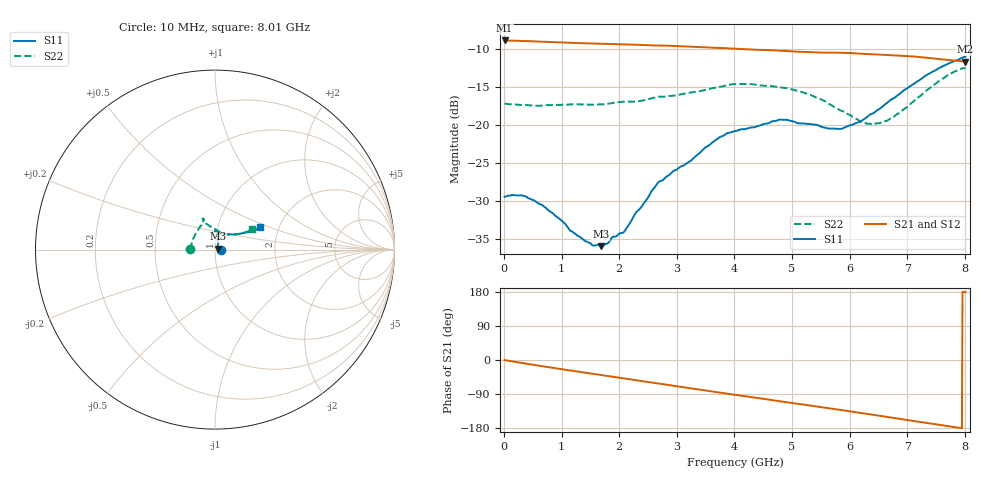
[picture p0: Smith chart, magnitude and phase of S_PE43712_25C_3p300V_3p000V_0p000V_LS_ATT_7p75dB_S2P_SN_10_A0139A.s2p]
! DEVICE ID: PE43712
! File Path: z:\PE43713\PE43713_CHAR_NOM_04292014\AMB\3p300\LS_ATT_7p75dB\PE43713_AMB_3p300V_3p000V_0p000V_LS_ATT_7p75dB_S2P_SN_10_A0139A.s2p
! Serial: 10
! Lot: A0139A
! Temp: 25C
! VDD: 3.300
! VSS: 0.000
! Control_Hi: 3.000
! Control_Lo: 0.000
! Attenuation Step: 7.75dB
! Port 1: RF1
! Port 2: RF2
! ThroughPath:1-2
! IDD: 0.0001474223
! ISS: -2.092e-007
#  Hz  S  RI  R  50
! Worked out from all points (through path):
!   801 points, 10 MHz to 8.01 GHz, reference 50 ohm
!   highest |S21| = -8.90 dB at 10 MHz (marker M1); lowest = -11.7 dB at 8.01 GHz (marker M2)
!   group delay of S21, straight-line fit = 62.2 ps
!   lowest |S11| = -35.9 dB at 1.68 GHz (marker M3), VSWR 1.03, Z = 51.5 + j0.548 ohm
!   |S11| at or under -10 dB: start of sweep to end of sweep
!   |S22| runs from -20.0 to -12.5 dB; largest |S21 - S12| = 0.0012
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1e7  0.0337 0.00011  0.3588 -0.0019  0.3588 -0.00189  -0.138 0.000826
3e8  0.0341 -0.00435  0.3531 -0.0474  0.353 -0.0474  -0.1345 0.0138
5.1e8  0.0315 -0.00604  0.3452 -0.0782  0.3452 -0.0781  -0.1319 0.0223
6.9e8  0.0284 -0.00621  0.3364 -0.1029  0.3364 -0.103  -0.1305 0.031
1.35e9  0.0179 -0.00129  0.2916 -0.1828  0.2917 -0.1829  -0.1227 0.059
1.55e9  0.0159 0.00231  0.2749 -0.2041  0.2749 -0.2041  -0.117 0.0688
1.68e9  0.015 0.00532  0.2634 -0.217  0.2634 -0.2171  -0.1143 0.0748
2.09e9  0.0133 0.0148  0.2231 -0.254  0.2231 -0.2539  -0.106 0.0942
2.68e9  0.0183 0.0379  0.1561 -0.293  0.1561 -0.293  -0.0822 0.1293
3.24e9  0.014 0.0563  0.0863 -0.3149  0.0864 -0.3149  -0.0707 0.1467
3.72e9  0.0117 0.081  0.0262 -0.3193  0.0259 -0.3193  -0.0657 0.1646
4.01e9  0.00784 0.0908  -0.00994 -0.3168  -0.00995 -0.3168  -0.0683 0.1723
4.79e9  0.00248 0.1083  -0.0993 -0.2909  -0.0993 -0.2911  -0.0638 0.1653
5.35e9  0.0139 0.0999  -0.1542 -0.2579  -0.1541 -0.2578  -0.0524 0.1467
5.63e9  0.0256 0.0912  -0.1786 -0.2391  -0.1785 -0.2392  -0.0341 0.1339
5.87e9  0.038 0.0864  -0.2004 -0.2201  -0.2001 -0.2202  -0.0146 0.1224
6.17e9  0.0606 0.0849  -0.2226 -0.1918  -0.2223 -0.192  0.0144 0.1051
6.33e9  0.0774 0.0854  -0.2328 -0.1765  -0.2323 -0.1764  0.0312 0.0969
6.68e9  0.1138 0.0861  -0.2509 -0.1397  -0.2505 -0.1398  0.069 0.0835
7.56e9  0.2126 0.1047  -0.2676 -0.0403  -0.2674 -0.0405  0.169 0.0974
7.81e9  0.2353 0.1153  -0.265 -0.0146  -0.2649 -0.0148  0.1955 0.1076
8.01e9  0.2522 0.1231  -0.2602 0.0042  -0.26 0.00373  0.2082 0.1122
